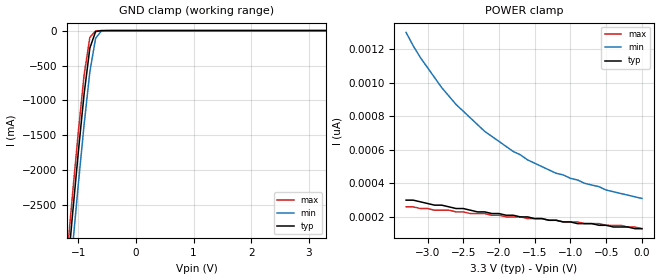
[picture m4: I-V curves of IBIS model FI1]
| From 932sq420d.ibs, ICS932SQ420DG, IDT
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|   Model FI1
[Model]   FI1
Model_type   Input
Polarity   Inverting
Enable   Active-High
Vinl =   0.80V
Vinh =   2.00V
C_comp   3.40pF   2.85pF   3.95pF
[Temperature Range]   27.00   70.00   0.000
[Voltage Range]   3.30V   3.00V   3.70V
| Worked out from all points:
|   GND clamp passes 1 mA (typ) near -0.60 V on its own axis
[GND_clamp]
| voltage   I(typ)   I(min)   I(max)
-3.3V     -24.05A    -24.48A    -23.79A
-1.2V     -3.55A     -4.02A     -3.26A
-1.1V     -2.63A     -3.1A      -2.34A
-1V       -1.74A     -2.2A      -1.45A
-900mV    -910mA     -1.35A     -640mA
-800mV    -250mA     -590mA     -96.82mA
-700mV    -14.58mA   -110mA     -3.87mA
-600mV    -880uA     -5.82mA    -450uA
-500mV    -88.5uA    -350uA     -45.09uA
3.3V      130pA      340pA      120pA
[POWER_clamp]
| voltage   I(typ)   I(min)   I(max)
-3.3V     300pA      1.3nA      260pA
-3.1V     290pA      1.15nA     250pA
-2.9V     270pA      1.03nA     240pA
-2.8V     270pA      970pA      240pA
-2.6V     250pA      870pA      230pA
-2.2V     230pA      710pA      220pA
-1.8V     210pA      590pA      200pA
-1.2V     180pA      460pA      180pA
-900mV    160pA      420pA      170pA
-500mV    150pA      360pA      150pA
-300mV    140pA      340pA      150pA
0V        130pA      310pA      130pA
